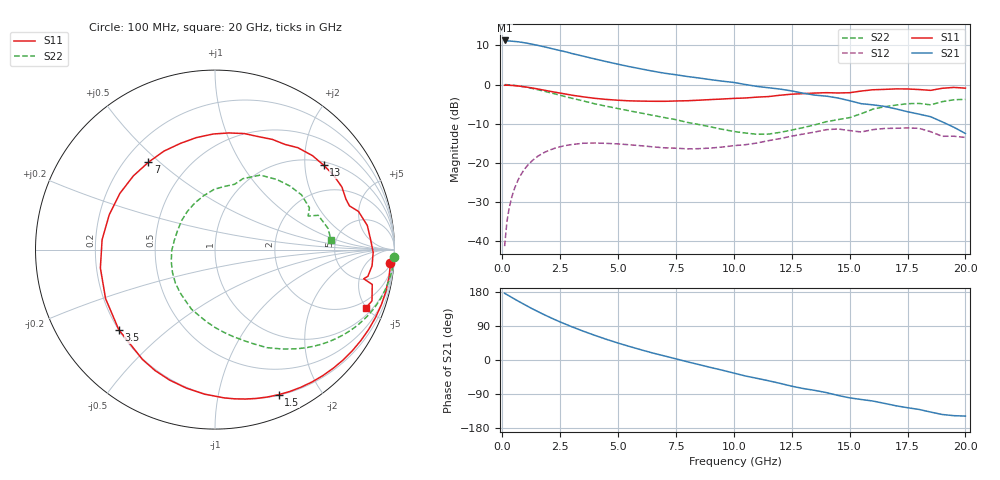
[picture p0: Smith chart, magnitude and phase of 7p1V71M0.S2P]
! Infineon Technologies  Discrete & RF Semiconductors
! bfp620
! VCE =  1.7 V,  IC =  1.0 mA
! Common Emitter S-Parameters:  Sep 2002
# GHz  S  MA  R  50
!  f  S11  S21  S12  S22
! GHz  MAG  ANG  MAG  ANG  MAG  ANG  MAG  ANG
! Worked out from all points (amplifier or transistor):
!   59 points, 100 MHz to 20 GHz, reference 50 ohm
!   highest |S21| = 11.3 dB at 100 MHz (marker M1)
!   |S21| within 3 dB of that: start of sweep to 2.808 GHz
!   unconditionally stable (mu >= 1): 6.341 GHz to 15.76 GHz; 17.84 GHz to end of sweep
!   at 1 GHz: K = 0.10, MSG = 15.9 dB, |S12| = -21.3 dB
!   at 5.5 GHz: K = 0.83, MSG = 10.0 dB, |S12| = -15.4 dB
!   at 20 GHz: K = 1.39, MAG = -3.2 dB, |S12| = -13.5 dB
!   S11 on the Smith chart (normalised r, x): 100 MHz: 6, -24; 1.5 GHz: 0.21, -1.51; 3.5 GHz: 0.20, -0.35; 7 GHz: 0.30, +0.46; 13 GHz: 1.10, +2.50; 20 GHz: 1.43, -4.94
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0.1  0.9805 -4.5  3.654 176.0  0.0087 87.6  0.9996 -2.4
0.2  0.9818 -9.1  3.62 172.5  0.0178 85.0  0.9962 -4.9
0.3  0.9802 -13.8  3.596 169.0  0.0269 82.4  0.9916 -7.3
0.5  0.9713 -22.9  3.557 161.9  0.0448 76.8  0.9789 -12.0
1  0.9332 -45.1  3.398 144.9  0.0864 62.0  0.9297 -23.0
1.5  0.8826 -66.3  3.178 128.9  0.1199 48.4  0.8649 -32.7
1.9  0.8386 -82.5  2.99 117.0  0.1401 38.7  0.8106 -39.6
2.4  0.788 -101.7  2.757 103.1  0.1584 28.0  0.7445 -47.3
3  0.7335 -123.4  2.493 87.8  0.172 16.7  0.6706 -55.7
3.5  0.6975 -140.2  2.303 76.0  0.1788 8.3  0.6182 -62.1
4  0.6681 -155.9  2.121 64.9  0.1799 0.6  0.5682 -67.6
5  0.6315 175.0  1.819 44.7  0.1752 -10.5  0.4945 -78.3
6  0.6157 149.5  1.584 26.8  0.1659 -18.6  0.4334 -90.1
7  0.612 127.3  1.398 10.8  0.1561 -22.8  0.3799 -103.1
8.5  0.6327 99.4  1.213 -12.2  0.1524 -24.7  0.3092 -129.0
10.5  0.6747 68.7  1.002 -42.2  0.1713 -27.8  0.2412 -178.7
13  0.7666 37.8  0.776 -75.3  0.2341 -39.5  0.2832 113.3
13.5  0.78 32.1  0.734 -80.2  0.2485 -44.1  0.3066 102.0
16  0.8591 9.0  0.552 -108.2  0.2664 -68.1  0.4858 58.7
17  0.8814 -1.0  0.49 -120.8  0.2774 -80.4  0.5477 40.2
18.5  0.844 -11.1  0.389 -137.4  0.2508 -103.7  0.5516 19.8
20  0.9005 -21.2  0.238 -148.0  0.2119 -109.5  0.6485 4.9
